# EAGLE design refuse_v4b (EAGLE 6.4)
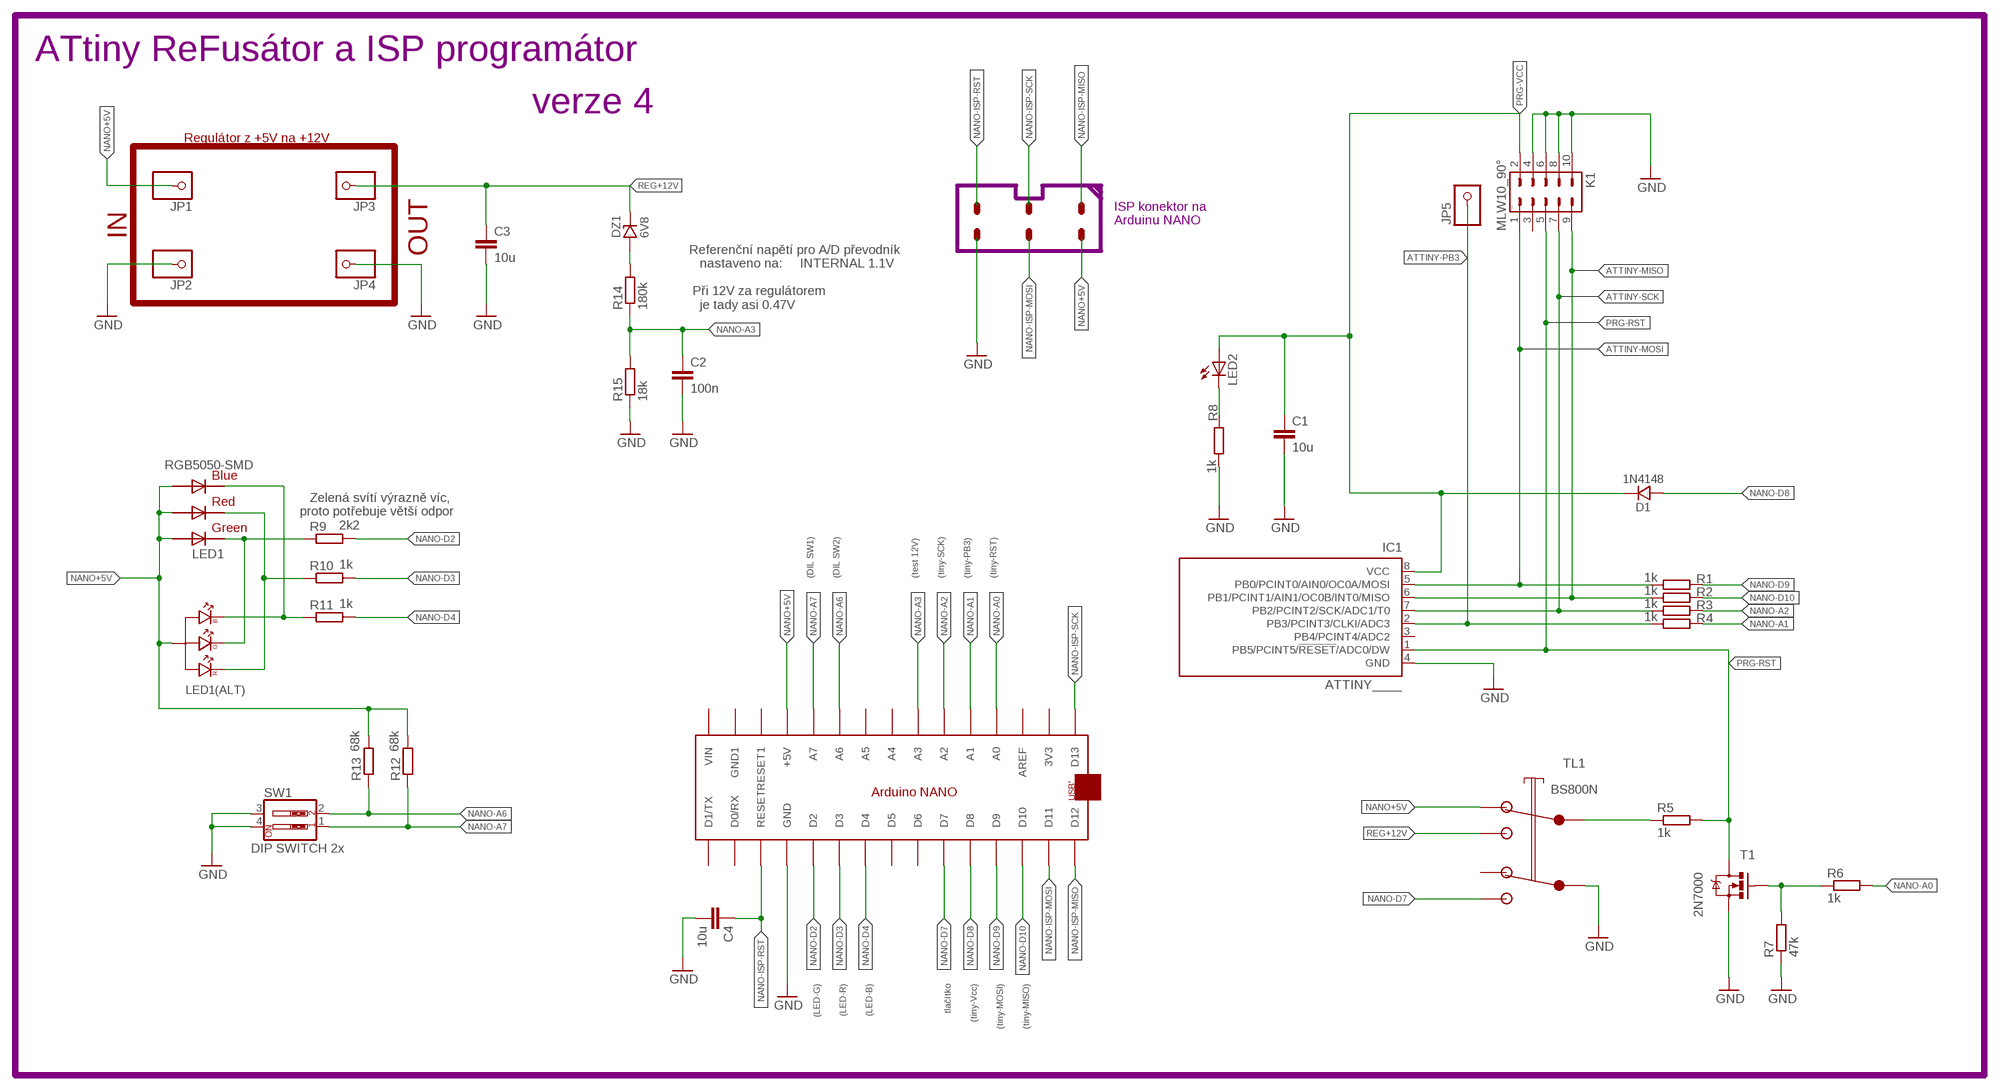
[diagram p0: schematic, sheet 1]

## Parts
ARDU1  Arduino NANO  ARDUINONANO  [PDIP-32]
C1  10u  C  [C0805]
C2  100n  C  [C0805]
C3  10u  C  [C0805]
C4  10u  C  [C0805]
D1  1N4148  1N4148.  [SOD-80]
DZ1  6V8  D-BZV55C_SMD_0,5W-ZENER  [SOD-80]
IC1  ATTINY____  TINY13-20PU  [DIL08]
JP1  pin  PINHD-1X1-BIGPOGO  [1X1-BIGPOGO]
JP2  pin  PINHD-1X1-BIGPOGO  [1X1-BIGPOGO]
JP3  pin  PINHD-1X1-BIGPOGO  [1X1-BIGPOGO]
JP4  pin  PINHD-1X1-BIGPOGO  [1X1-BIGPOGO]
JP5  pin  PINHD-1X1-BIGPOGO  [1X1-BIGPOGO]
K1  MLW10_90°  [MLW10A]
LED1  RGB5050-SMD  RGBLED5050  [RGBLED5050]
LED1(ALT)  RGB LED - THT  LED_RGB  [LED_5-RGB]
LED2  SMD 0805  LEDCHIPLED_0805  [CHIPLED_0805]
R1  1k  R-EU_M0805  [M0805]
R2  1k  R-EU_M0805  [M0805]
R3  1k  R-EU_M0805  [M0805]
R4  1k  R-EU_M0805  [M0805]
R5  1k  R-EU_M0805  [M0805]
R6  1k  R-EU_M0805  [M0805]
R7  47k  R-EU_M0805  [M0805]
R8  1k  R-EU_M0805  [M0805]
R9  2k2  R-EU_M0805  [M0805]
R10  1k  R-EU_M0805  [M0805]
R11  1k  R-EU_M0805  [M0805]
R12  68k  R-EU_M0805  [M0805]
R13  68k  R-EU_M0805  [M0805]
R14  180k  R-EU_M0805  [M0805]
R15  18k  R-EU_M0805  [M0805]
SW1  DIP SWITCH 2x  SW_DIP-2  [EDG-02]
T1  2N7000  MOSFET-NCHANNELPTH  [TO-92]
TL1  BS800N  BUTTON2X  [8X8-DPDT]

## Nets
ATTINY-MISO: IC1.6(PB1/PCINT1/AIN1/OC0B/INT0/MISO) K1.9 R2.1
ATTINY-MOSI: IC1.5(PB0/PCINT0/AIN0/OC0A/MOSI) K1.1 R1.1
ATTINY-PB3: IC1.2(PB3/PCINT3/CLKI/ADC3) JP5.P$1 R4.1
ATTINY-SCK: IC1.7(PB2/PCINT2/SCK/ADC1/T0) K1.7 R3.1
GATE: R6.1 R7.2 T1.3(G)
GND: ARDU1.GND C1.2 C2.2 C3.2 C4.2 IC1.4(GND) JP2.P$1 JP4.P$1 K1.4 K1.6 K1.8 K1.10 R7.1 R8.1 R15.1 SW1.3 SW1.4 T1.1(S) TL1.X2(COM2)
LEDBLU: LED1(ALT).4(B) LED1.6(BLUE_C) R11.1
LEDGRN: LED1(ALT).3(G) LED1.4(GREEN_C) R9.1
LEDRED: LED1(ALT).1(R) LED1.5(RED_C) R10.1
N$2: LED2.C R8.2
N$6: DZ1.A R14.2
NANO+5V: ARDU1.+5V JP1.P$1 LED1(ALT).2(A) LED1.1(BLUE_A) LED1.2(RED_A) LED1.3(GREEN_A) R12.2 R13.2 TL1.C1(NC1)
NANO-A0: ARDU1.A0 R6.2
NANO-A1: ARDU1.A1 R4.2
NANO-A2: ARDU1.A2 R3.2
NANO-A3: ARDU1.A3 C2.1 R14.1 R15.2
NANO-A6: ARDU1.A6 R13.1 SW1.2
NANO-A7: ARDU1.A7 R12.1 SW1.1
NANO-D2: ARDU1.D2 R9.2
NANO-D3: ARDU1.D3 R10.2
NANO-D4: ARDU1.D4 R11.2
NANO-D7: ARDU1.D7 TL1.O2(NO2)
NANO-D8: ARDU1.D8 D1.A
NANO-D9: ARDU1.D9 R1.2
NANO-D10: ARDU1.D10 R2.2
NANO-ISP-MISO: ARDU1.D12
NANO-ISP-MOSI: ARDU1.D11
NANO-ISP-RST: ARDU1.RESET C4.1
NANO-ISP-SCK: ARDU1.D13
PRG-RST: IC1.1(PB5/PCINT5/!RESET!/ADC0/DW) K1.5 R5.2 T1.2(D)
PRG-VCC: C1.1 D1.K IC1.8(VCC) K1.2 LED2.A
REG+12V: C3.1 DZ1.K JP3.P$1 TL1.O1(NO1)
TL1-COM: R5.1 TL1.X1(COM1)
Unconnected: ARDU1.3V3 ARDU1.A4 ARDU1.A5 ARDU1.AREF ARDU1.D0/RX ARDU1.D1/TX ARDU1.D5 ARDU1.D6 ARDU1.GND1 ARDU1.RESET1 ARDU1.VIN IC1.3(PB4/PCINT4/ADC2) K1.3 TL1.C2(NC2)

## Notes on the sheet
- ATtiny ReFusátor a ISP programátor
- verze 4
- Regulátor z +5V na +12V
- OUT
- IN
- ISP konektor na 
  Arduinu NANO
- Referenční napětí pro A/D převodník
     nastaveno na:     INTERNAL 1.1V
  
   Při 12V za regulátorem
     je tady asi 0.47V
- Zelená svítí výrazně víc, 
  proto potřebuje větší odpor
- (DIL SW1) | (DIL SW2) | (test 12V) | (tiny-SCK) | (tiny-PB3) | (tiny-RST)
- Arduino NANO
- (LED-G) | (LED-R) | (LED-B) | tlačítko | (tiny-Vcc) | (tiny-MOSI) | (tiny-MISO)

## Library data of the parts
ARDU1 = jet-lib:ARDUINONANO
C1-C4 = eagle-ltspice:C: CAPACITOR, European symbol; SPICEMODEL: NONE; SPICEPREFIX: C
D1 = #PaJa_31:1N4148: Univerzalni dioda - 0,15A, 75V
DZ1 = #PaJa_31:D-?-ZENER: Zenerova dioda
IC1 = atmel:TINY13: 8-bit AVR Microcontroller with 1K Bytes In-System Programmable Flash Source: http://www.atmel.com/dyn/resources/prod_documents/2535S.pdf; MPN: ATTINY13-20PU; OC_FARNELL: 9171550; OC_NEWARK: 96K6521
JP1-JP5 = adafruit:PINHD-1X1: Pin header 1x1 for 0.1" spacing
K1 = #PaJa_konektory:MLW10: Konektory MLW - vidlice - 10x
LED1 = adafruit:RGBLED: For 5050 RGB LEDs, the order of the LEDs may vary from one manufacturer to another!
LED1(ALT) = #PaJa_31:LED_RGB: LED dioda - RGB - trojbarevna - 4 vyvody, spol. Anoda
LED2 = led:LED: LED
R1-R15 = resistor:R-EU_: RESISTOR, European symbol
SW1 = special:SW_DIP-2: DIP SWITCH
T1 = 2n7000:MOSFET-NCHANNEL
TL1 = tlacitko2x:BUTTON2X: Dvojite prepinaci tlacitko; 1 stabilni poloha; 8x8mm; BS800N

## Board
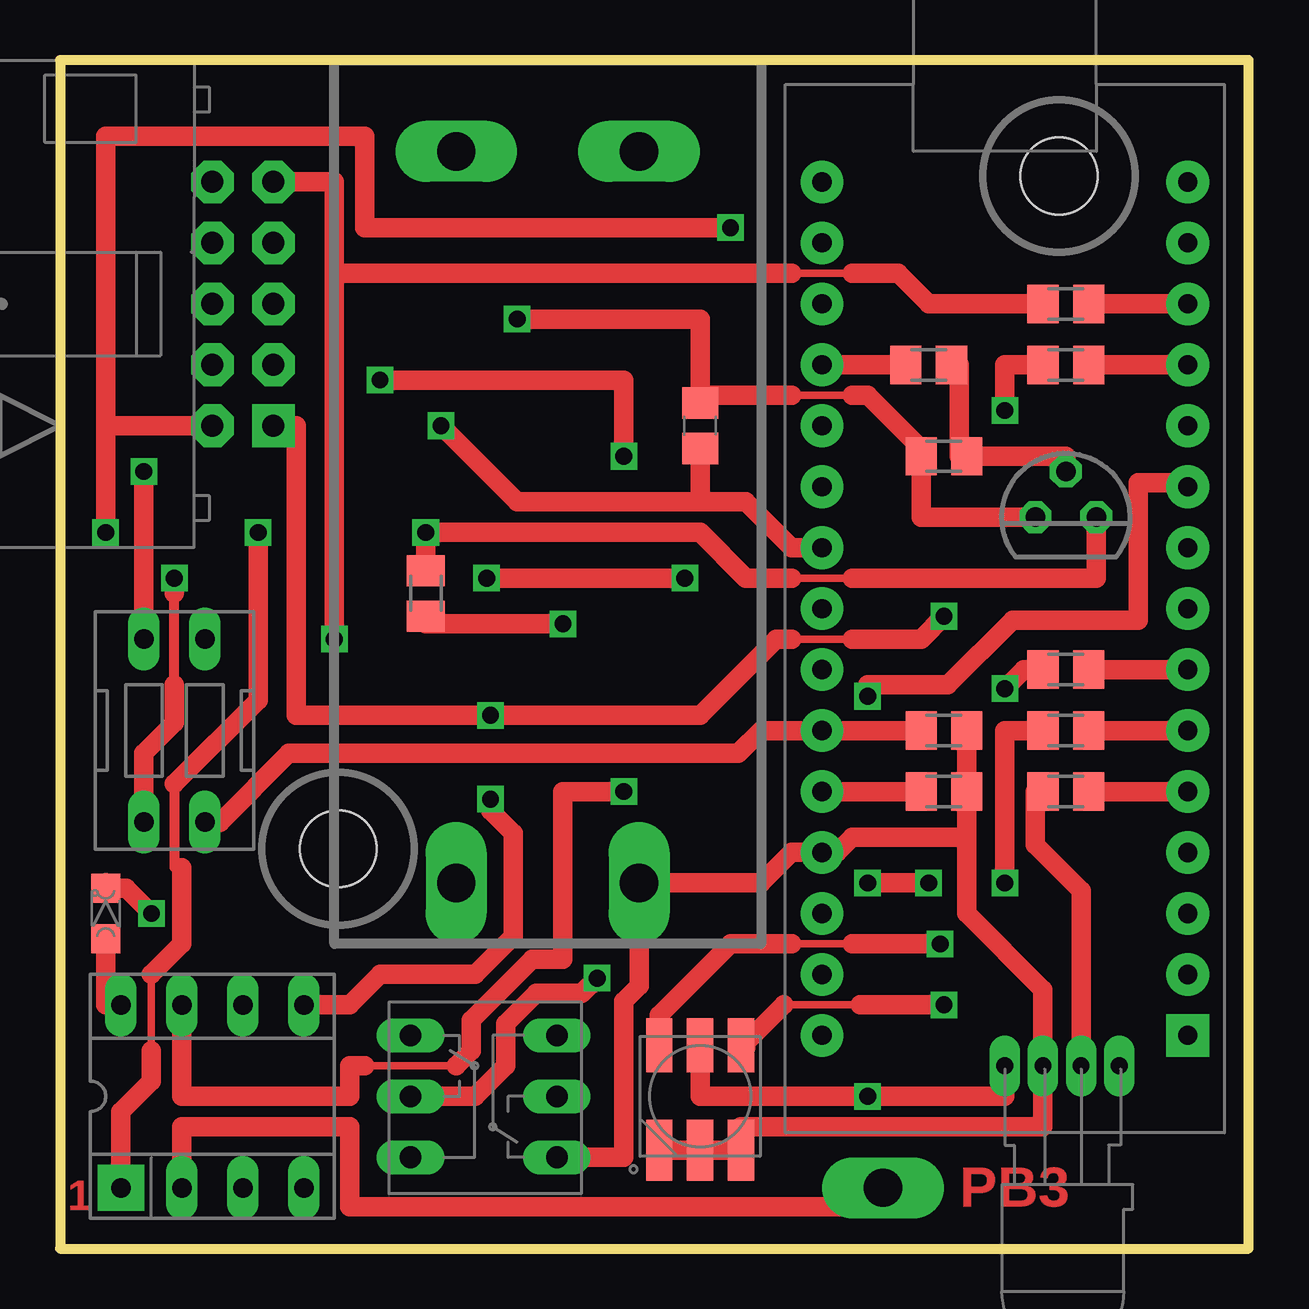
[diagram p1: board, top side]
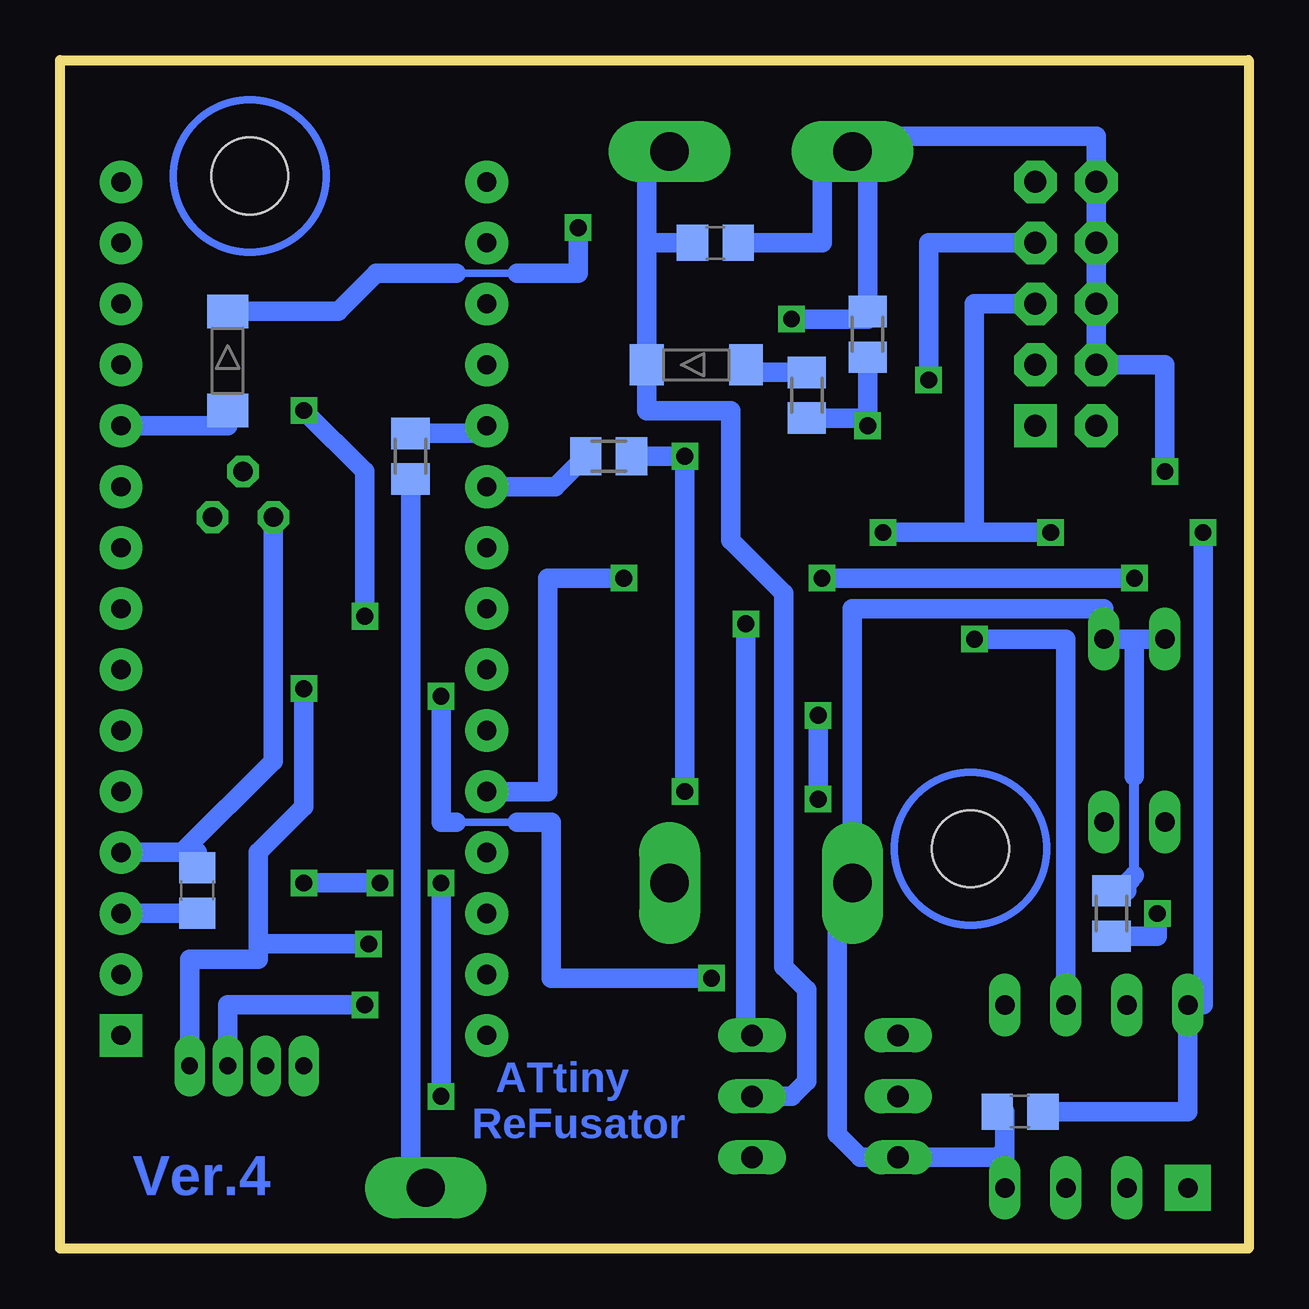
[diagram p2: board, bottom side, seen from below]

Size 49.53 x 49.53 mm. Coordinates in mm from the lower left corner, seen from the top.
Outline: 0,0 49.53,0 49.53,49.53 0,49.53 0,0
Copper layers (1*16): Top 0.035mm / dielectric 1.5mm / Bottom 0.035mm
Design rules "default *": minimum track width 10mil, minimum drill 24mil, track to track 8mil, track to pad 8mil, pad to pad 8mil, via to via 8mil, smd to smd 8mil, copper to edge 40mil, drill to drill 8mil, minimum pad ring 10mil, minimum via ring 8mil, stop-mask expansion 4mil, vias tented up to drill 0mil, thermal gap 10mil
Holes 3.2 mm at 41.62,44.7 11.59,16.67

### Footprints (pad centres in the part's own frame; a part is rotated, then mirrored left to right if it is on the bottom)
PDIP-32 = drill 0.8 pad 1.778: 3V3 15.24,-35.56; +5V 15.24,-10.16; A0 15.24,-30.48; A1 15.24,-27.94; A2 15.24,-25.4; A3 15.24,-22.86; A4 15.24,-20.32; A5 15.24,-17.78; A6 15.24,-15.24; A7 15.24,-12.7; AREF 15.24,-33.02; D0/RX 0,-5.08; D2 0,-12.7; D3 0,-15.24; D4 0,-17.78; D5 0,-20.32; D6 0,-22.86; D7 0,-25.4; D8 0,-27.94; D9 0,-30.48; D10 0,-33.02; D11 0,-35.56; D12 0,-38.1; D13 15.24,-38.1; GND 0,-10.16; GND1 15.24,-5.08; RESET 0,-7.62; RESET1 15.24,-7.62; VIN 15.24,-2.54 | drill 0.8 pad 1.778 square: D1/TX 0,-2.54
C0805 = smd 1.3 x 1.5: 1 -0.95,0; 2 0.95,0
SOD-80 = smd 1.397 x 1.702: A 1.905,0; K -2.223,0
DIL08 = drill 0.813 pad 1.93 square: 1 -3.81,-3.81 | drill 0.813 long: 2 -1.27,-3.81; 3 1.27,-3.81; 4 3.81,-3.81; 5 3.81,3.81; 6 1.27,3.81; 7 -1.27,3.81; 8 -3.81,3.81
1X1-BIGPOGO = drill 1.6 pad 2.54 long: P$1 0,0
MLW10A = drill 0.914 pad 1.778 square: 1 -5.08,-1.27 | drill 0.914 pad 1.778 octagon: 2 -5.08,1.27; 3 -2.54,-1.27; 4 -2.54,1.27; 5 0,-1.27; 6 0,1.27; 7 2.54,-1.27; 8 2.54,1.27; 9 5.08,-1.27; 10 5.08,1.27
RGBLED5050 = smd 2.54 x 1.1: 1 -2.254,1.7; 2 -2.254,0; 3 -2.254,-1.7 | smd 2.254 x 1.1: 4 2.127,-1.7; 5 2.127,0; 6 2.127,1.7
LED_5-RGB = drill 0.7 pad 1.27 long: 1 -2.54,0; 2 -0.953,0; 3 0.635,0; 4 2.223,0
CHIPLED_0805 = smd 1.2 x 1.2: A 0,-1.05; C 0,1.05
M0805 = smd 1.3 x 1.6: 1 -0.95,0; 2 0.95,0
EDG-02 = drill 0.813 long: 1 -1.27,-3.81; 2 1.27,-3.81; 3 1.27,3.81; 4 -1.27,3.81
TO-92 = drill 0.813 octagon: 1 -1.27,0; 2 1.27,0; 3 0,1.905
8X8-DPDT = drill 0.9 pad 1.27 long: C1 2.54,2.921; C2 -2.54,-3.175; O1 0,2.921; O2 0,-3.175; X1 -2.54,2.921; X2 2.54,-3.175

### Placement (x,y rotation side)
ARDU1  46.99,6.35 180 top
C1  9.53,5.71 180 bottom
C2  26.67,34.29 90 top
C3  22.23,41.91 0 bottom
C4  43.81,14.92 90 bottom
D1  42.55,36.83 270 bottom
DZ1  22.86,36.83 0 bottom
IC1  6.35,6.35 0 top
JP1  24.13,15.24 270 top
JP2  16.51,15.24 270 top
JP3  24.13,45.72 180 top
JP4  16.51,45.72 180 top
JP5  34.29,2.54 0 top
K1  7.62,39.37 90 top
LED1  26.67,6.35 90 top
LED1(ALT)  41.91,7.62 0 top
LED2  1.91,13.97 0 top
R1  41.91,36.83 0 top
R2  41.91,39.37 0 top
R3  26.67,33.02 180 bottom
R4  34.92,33.02 90 bottom
R5  15.24,27.3 90 top
R6  36.2,36.83 180 top
R7  36.83,33.02 0 top
R8  5.71,13.97 270 bottom
R9  41.91,19.05 0 top
R10  41.91,21.59 0 top
R11  41.91,24.13 0 top
R12  36.83,19.05 0 top
R13  36.83,21.59 0 top
R14  18.41,35.56 90 bottom
R15  15.88,38.1 270 bottom
SW1  4.76,21.59 0 top
T1  41.91,30.48 0 top
TL1  17.78,6.35 270 top

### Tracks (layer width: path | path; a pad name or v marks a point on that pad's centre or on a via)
ATTINY-MISO  (via drill 0.7)
  Top 0.305: 33.02,40.64 30.48,40.64
  Top 0.813: R2.1 36.2,39.37 34.92,40.64 33.02,40.64 | 30.48,40.64 11.43,40.64 | 11.43,40.64 11.43,44.45 K1.9 | 11.43,40.64 v11.43,25.4
  Bottom 0.813: v11.43,25.4 7.62,25.4 IC1.6 7.62,9.53
ATTINY-MOSI  (via drill 0.7)
  Top 0.305: 30.48,25.4 33.02,25.4
  Top 0.813: K1.1 9.84,34.29 9.84,22.23 v17.94,22.23 26.67,22.23 29.84,25.4 30.48,25.4 | 33.02,25.4 35.88,25.4 v36.83,26.35 | v39.37,34.92 39.37,36.83 R1.1 | IC1.5 12.06,10.16 13.34,11.43 17.3,11.43 18.89,13.02 18.89,17.3 17.94,18.26 v17.94,18.73
  Bottom 0.813: v36.83,26.35 36.83,32.38 v39.37,34.92 | v17.94,18.73 v17.94,22.23
ATTINY-PB3
  Top 0.813: IC1.2 5.08,5.08 12.06,5.08 12.06,1.75 33.02,1.75 33.02,2.54 JP5.P$1
  Bottom 0.813: R4.1 34.92,2.54 JP5.P$1
ATTINY-SCK  (via drill 0.7)
  Top 0.305: 12.7,7.62 16.51,7.62
  Top 0.813: IC1.7 5.08,6.35 12.06,6.35 12.06,7.62 12.7,7.62 | v13.34,36.2 23.5,36.2 v23.5,33.02 | 16.51,7.62 17.14,8.26 17.14,9.53 19.68,12.06 20.95,12.06 20.95,19.05 v23.5,19.05
  Bottom 0.813: v23.5,19.05 v23.5,33.02 R3.1 | K1.7 13.34,41.91 v13.34,36.2
GATE
  Top 0.813: R6.1 37.47,36.83 37.47,33.02 R7.2 41.91,33.02 T1.3
GND  (via drill 0.7)
  Top 0.305: 33.02,35.56 30.48,35.56
  Top 0.813: T1.1 35.88,30.48 R7.1 35.88,33.34 33.66,35.56 33.02,35.56 | 30.48,35.56 26.67,35.56 | 26.67,35.56 26.67,38.73 v19.05,38.73 | SW1.4 v3.49,32.38 | C2.2 26.67,35.56
  Bottom 0.406: 4.76,15.24 4.76,15.56 4.76,19.68
  Bottom 0.813: JP4.P$1 15.88,45.72 R15.1 15.88,38.73 v19.05,38.73 | JP4.P$1 16.51,46.35 6.35,46.35 K1.10 K1.8 K1.6 K1.4 3.49,36.83 v3.49,32.38 | SW1.4 4.76,25.4 | 4.76,25.4 SW1.3 6.03,26.67 16.51,26.67 JP2.P$1 | JP2.P$1 17.14,15.24 | T1.1 40.64,20.32 44.45,16.51 ARDU1.GND 43.81,16.51 C4.2 | C1.2 10.16,5.71 10.16,4.13 | 10.16,4.13 IC1.4 | C3.2 17.78,41.91 17.78,45.72 JP4.P$1 | R8.1 5.08,14.92 5.08,15.24 4.76,15.56 | 4.76,19.68 4.76,25.4 | 10.16,4.13 10.48,3.81 TL1.X2 16.19,3.81 17.14,4.76 17.14,14.61 JP2.P$1
LEDBLU  (via drill 0.7)
  Top 0.305: 30.48,12.7 33.02,12.7
  Top 0.813: 30.48,12.7 27.94,12.7 24.97,9.73 LED1.6 | 33.02,12.7 v36.67,12.7 | v39.37,23.34 40.16,24.13 R11.1
  Bottom 0.813: 41.27,12.7 41.27,16.51 39.37,18.41 v39.37,23.34 | v36.67,12.7 41.27,12.7 | LED1(ALT).4 44.13,12.06 41.27,12.06 41.27,12.7
LEDGRN  (via drill 0.7)
  Top 0.305: 30.16,10.16 33.34,10.16
  Top 0.813: R9.1 40.64,19.05 40.64,16.83 42.55,14.92 LED1(ALT).3 | 28.37,8.37 30.16,10.16 | 33.34,10.16 v36.83,10.16 | 28.37,8.37 28.57,8.37 28.57,9.05 28.37,9.05 | 28.37,8.37 LED1.4
  Bottom 0.813: v36.83,10.16 42.55,10.16 LED1(ALT).3
LEDRED  (via drill 0.7)
  Top 0.813: R10.1 39.37,21.59 v39.37,15.24 | v36.2,15.24 v33.66,15.24 | LED1.5 26.67,6.35 29.53,6.35 v33.66,6.35 39.37,6.35 LED1(ALT).1
  Bottom 0.813: v39.37,15.24 v36.2,15.24 | v33.66,6.35 v33.66,15.24
N$2  (via drill 0.7)
  Top 0.813: 1.91,15.24 LED2.C 2.76,15.02 v3.81,13.97
  Bottom 0.813: R8.2 3.81,13.02 v3.81,13.97
N$6
  Bottom 0.813: R14.2 20.95,36.51 DZ1.A
NANO+5V
  Top 0.813: R13.2 R12.2 37.78,17.14 | 37.78,17.14 37.78,13.97 40.96,10.79 LED1(ALT).2 40.96,5.08 28.37,5.08 LED1.3 LED1.2 LED1.1 | 37.78,17.14 33.02,17.14 32.38,16.51 ARDU1.+5V 30.48,16.51 29.21,15.24 JP1.P$1 24.13,10.95 23.5,10.32 23.5,3.81 TL1.C1
NANO-A0
  Top 0.813: R6.2 ARDU1.A0
NANO-A1
  Bottom 0.813: ARDU1.A1 31.75,33.97 R4.2
NANO-A2
  Bottom 0.813: ARDU1.A2 28.89,31.75 R3.2
NANO-A3  (via drill 0.7)
  Top 0.813: 26.67,31.11 28.57,31.11 30.48,29.21 ARDU1.A3 | 26.67,31.11 19.05,31.11 v15.88,34.29 | C2.1 26.67,31.11
  Bottom 0.813: 15.88,34.61 R15.2 | R14.1 15.88,34.61 | 15.88,34.61 v15.88,34.29
NANO-A6
  Top 0.813: R13.1 ARDU1.A6 29.21,21.59 28.26,20.64 9.53,20.64 6.67,17.78 SW1.2
NANO-A7  (via drill 0.7)
  Top 0.406: 4.76,23.5 4.76,27.3
  Top 0.813: R12.1 ARDU1.A7 | SW1.1 3.49,20.64 4.76,21.91 4.76,23.5 | 4.76,27.3 v4.76,27.94 | v17.78,27.94 v26.04,27.94
  Bottom 0.813: v4.76,27.94 v17.78,27.94 | ARDU1.A7 29.21,19.05 29.21,27.94 v26.04,27.94
NANO-D2
  Top 0.813: R9.2 ARDU1.D2
NANO-D3
  Top 0.813: R10.2 ARDU1.D3
NANO-D4
  Top 0.813: R11.2 ARDU1.D4
NANO-D7  (via drill 0.7)
  Top 0.813: TL1.O2 17.3,6.35 18.57,7.62 18.57,9.37 19.84,10.64 21.75,10.64 v22.38,11.27 | v33.66,23.02 33.66,23.5 36.99,23.5 39.69,26.19 44.93,26.19 44.93,31.91 46.99,31.91 ARDU1.D7
  Bottom 0.305: 33.02,17.78 30.48,17.78
  Bottom 0.813: v22.38,11.27 29.05,11.27 29.05,17.78 30.48,17.78 | v33.66,23.02 33.66,17.78 33.02,17.78
NANO-D8
  Bottom 0.813: ARDU1.D8 42.55,34.29 D1.A
NANO-D9
  Top 0.813: R1.2 ARDU1.D9
NANO-D10
  Top 0.813: R2.2 ARDU1.D10
NANO-ISP-RST
  Bottom 0.813: ARDU1.RESET C4.1
PRG-RST  (via drill 0.7)
  Top 0.305: 3.81,11.43 3.81,8.26 | 33.02,27.94 30.48,27.94
  Top 0.406: 4.76,19.37 4.76,15.88 5.08,15.88
  Top 0.813: v8.26,29.84 8.26,22.86 4.76,19.37 | 3.81,8.26 3.81,6.99 2.54,5.71 IC1.1 | T1.2 43.18,27.94 33.02,27.94 | R5.2 v15.24,29.84 26.67,29.84 28.57,27.94 30.48,27.94 | 5.08,15.88 5.08,12.7 3.81,11.43
  Bottom 0.813: K1.5 11.43,39.37 11.43,29.84 | v15.24,29.84 11.43,29.84 | 11.43,29.84 v8.26,29.84
PRG-VCC  (via drill 0.7)
  Top 0.813: v1.91,29.84 1.91,34.29 | LED2.A 1.91,10.16 IC1.8 | 1.91,34.29 1.91,46.35 12.7,46.35 12.7,42.55 v27.94,42.55 | K1.2 1.91,34.29
  Bottom 0.305: 33.02,40.64 30.48,40.64
  Bottom 0.813: v1.91,29.84 1.91,10.16 IC1.8 2.54,5.71 C1.1 | D1.K 37.94,39.05 36.35,40.64 33.02,40.64 | 30.48,40.64 27.94,40.64 v27.94,42.55
REG+12V
  Bottom 0.813: JP3.P$1 25.08,45.72 25.08,41.91 | 25.08,41.91 DZ1.K 25.08,34.92 21.59,34.92 21.59,29.53 19.37,27.3 19.37,11.75 18.41,10.79 18.41,6.99 19.05,6.35 TL1.O1 | C3.1 25.08,41.91
TL1-COM  (via drill 0.7)
  Top 0.813: R5.1 15.24,26.04 v20.95,26.04
  Bottom 0.813: TL1.X1 20.95,8.89 v20.95,26.04
(copper drawn outside any net)
  shapes: Bottom circle x2, Top circle x2

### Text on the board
Top: 1 | PB3
Bottom: ATtiny / ReFusator | Ver.4
tDocu: 10 9 | GND | +12V / (OUT) | 2 1 | GND | +5V / (IN) | PB3 | Pozor: / Některé RGB SMD LED mají značku u katody. / Osaďte LED podle popisků.
bDocu: G | S | D
topvaldoc: Step-Up regul. / 5V -> 12V | 2x 1k | 2x 68k | 2k2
